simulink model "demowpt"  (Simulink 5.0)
settings: Solver=ode45  StartTime=0.0  StopTime=50  MaxStep=10^-2  RelTol=1e-3
libraries: simulink x3, MarineGNC x1

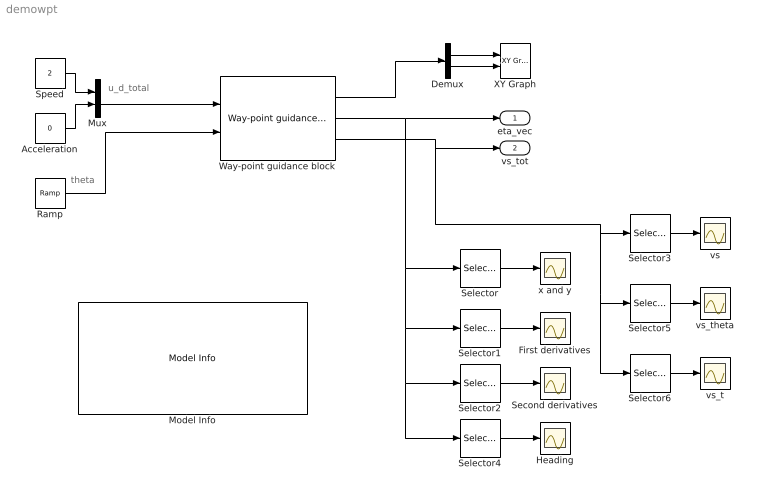
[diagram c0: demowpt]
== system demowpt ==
  note: u_d_total
  note: theta
  Acceleration : Constant  Value=0
  Demux : Demux  Outputs=2
  First derivatives : Scope
  Heading : Scope
  Model Info : simulink/Model-Wide Utilities/Model Info  InitialBlockCM=None  BlockCM=None  Frame=on  DisplayStringWithTags=|  HorizontalTextAlignment=Left  LeftAlignmentValue=0.02  SourceBlockDiagram=demowpt  TagMaxNumber=20
      | Way-point Guidance Demo.
      | Creates a 3 times differentiable path between 
      | the provided way-points. The user can choose
      | between cubic splines (3rd order)  and a 5th
      | order polynomial.
      | Author: Jørgen Corneliussen
      | %<ModifiedDate>
  Mux : Mux  Inputs=2
  Ramp : simulink/Sources/Ramp  slope=1  start=0  X0=0
  Second derivatives : Scope
  Selector : Selector  Elements=[1 2]  InputPortWidth=9
  Selector1 : Selector  Elements=[4 5]  InputPortWidth=9
  Selector2 : Selector  Elements=[7 8]  InputPortWidth=9
  Selector3 : Selector  InputPortWidth=3
  Selector4 : Selector  Elements=3  InputPortWidth=9
  Selector5 : Selector  Elements=2  InputPortWidth=3
  Selector6 : Selector  Elements=3  InputPortWidth=3
  Speed : Constant  Value=2
  Way-point guidance block : MarineGNC/Guidance/Way-point guidance block  x_vector=[-800 -500 -200 -50 -200 -250 200 500 500 300 0 -300 -600]  y_vector=[100 1800 2000 1500 1000 100 1000 300 -250 -200 100 -600 -1000]  method=5th order polynomial  drawmode=on  stop=on  mode=Acc  start=[100 0]  final=[0 100]  constraint=off
  XY Graph : simulink/Sinks/XY Graph  xmin=-3000  xmax=3000  ymin=-3000  ymax=3000  st=-1
  vs : Scope
  vs_t : Scope
  vs_theta : Scope
  x and y : Scope
  eta_vec : Outport
  vs_tot : Outport  Port=2
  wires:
  Speed/1 -> Mux/1
  Acceleration/1 -> Mux/2
  Mux/1 -> Way-point guidance block/1
  Way-point guidance block/2 -> eta_vec/1, Selector/1, Selector1/1, Selector2/1, Selector4/1
  Ramp/1 -> Way-point guidance block/2
  Way-point guidance block/3 -> vs_tot/1, Selector3/1, Selector6/1, Selector5/1
  Selector/1 -> x and y/1
  Selector1/1 -> First derivatives/1
  Selector2/1 -> Second derivatives/1
  Way-point guidance block/1 -> Demux/1
  Selector3/1 -> vs/1
  Selector4/1 -> Heading/1
  Selector5/1 -> vs_theta/1
  Selector6/1 -> vs_t/1
  Demux/1 -> XY Graph/1
  Demux/2 -> XY Graph/2
